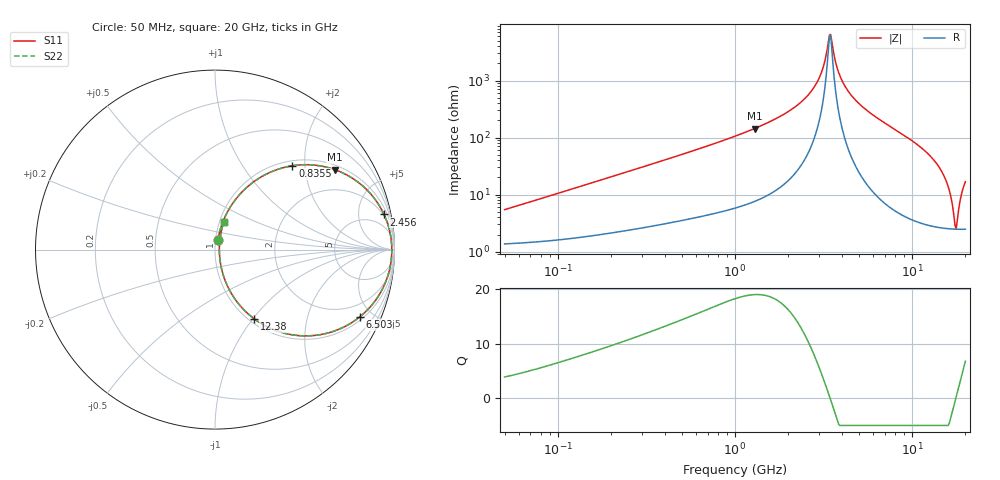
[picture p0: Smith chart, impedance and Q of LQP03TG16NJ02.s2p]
!Murata Part Number: LQP03TG16NJ02
!These Parameters are Measured in Series Mode Connection
!  o--[Z]--o
!Port1  Port2
!  o-------o
!Freq. Start=50[MHz] Stop=20[GHz], 401[Steps]
# Hz S RI R 50
!Freq.(Hz) S11(Real) S11(Imag) S21(Real) S21(Imag) S12(Real) S12(Imag) S22(Real) S22(Imag)
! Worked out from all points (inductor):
!   401 points, 50 MHz to 20 GHz, reference 50 ohm
!   read as one part in series: L = 16.7 nH near 51.52 MHz
!   highest Q = 19 at 1.29 GHz (marker M1), where L = 17.8 nH
!   self-resonance near 3.415 GHz
!   S11 on the Smith chart (normalised r, x): 50 MHz: 1.03, +0.11; 835.5 MHz: 1.10, +1.73; 2.456 GHz: 1.79, +9.37; 6.503 GHz: 1.17, -4.21; 12.38 GHz: 1.06, -1.02; 20 GHz: 1.05, +0.33
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5e7  0.0162 0.0514  0.9838 -0.0514  0.9838 -0.0514  0.0162 0.0514
1.364002e8  0.0361 0.1335  0.9639 -0.1335  0.9639 -0.1335  0.0361 0.1335
3.721004e8  0.1427 0.3127  0.8573 -0.3127  0.8573 -0.3127  0.1427 0.3127
8.354841e8  0.4317 0.4672  0.5683 -0.4672  0.5683 -0.4672  0.4317 0.4672
1e9  0.5268 0.4726  0.4732 -0.4726  0.4732 -0.4726  0.5268 0.4726
1.289994e9  0.6676 0.4455  0.3324 -0.4455  0.3324 -0.4455  0.6676 0.4455
2.456456e9  0.9416 0.196  0.0584 -0.196  0.0584 -0.196  0.9416 0.196
2.728004e9  0.9639 0.1379  0.0361 -0.1379  0.0361 -0.1379  0.9639 0.1379
3.075291e9  0.9799 0.0682  0.0201 -0.0682  0.0201 -0.0682  0.9799 0.0682
3.364474e9  0.9849 0.0142  0.0151 -0.0142  0.0151 -0.0142  0.9849 0.0142
3.466789e9  0.9852 -0.00403  0.0148 0.00403  0.0148 0.00403  0.9852 -0.00403
3.792786e9  0.9819 -0.0592  0.0181 0.0592  0.0181 0.0592  0.9819 -0.0592
4.212059e9  0.9695 -0.1241  0.0305 0.1241  0.0305 0.1241  0.9695 -0.1241
6.503449e9  0.8061 -0.3753  0.1939 0.3753  0.1939 0.3753  0.8061 -0.3753
7.442007e9  0.7128 -0.4339  0.2872 0.4339  0.2872 0.4339  0.7128 -0.4339
1.238412e10  0.2193 -0.3864  0.7807 0.3864  0.7807 0.3864  0.2193 -0.3864
1.550395e10  0.0538 -0.1653  0.9462 0.1653  0.9462 0.1653  0.0538 -0.1653
1.646126e10  0.033 -0.0909  0.967 0.0909  0.967 0.0909  0.033 -0.0909
1.747767e10  0.0244 -0.0141  0.9756 0.0141  0.9756 0.0141  0.0244 -0.0141
1.800918e10  0.0248 0.0245  0.9752 -0.0245  0.9752 -0.0245  0.0248 0.0245
1.912117e10  0.0346 0.1004  0.9654 -0.1004  0.9654 -0.1004  0.0346 0.1004
2e10  0.0495 0.1552  0.9505 -0.1552  0.9505 -0.1552  0.0495 0.1552
